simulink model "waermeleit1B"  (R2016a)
settings: Solver=ode45  StartTime=0.0  StopTime=2000  MaxStep=0.2  RelTol=1e-3
InitFcn:
  | init_waermeleit1
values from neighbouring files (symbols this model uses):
  dx = L/N    (= 0.2)    [init_waermeleit1.m]
  kappa = 1.1632e-04    (= 0.00011632)    [init_waermeleit1.m]
  T0 = 500    [init_waermeleit1.m]
  Tl = 300    [init_waermeleit1.m]
  Tr = 250    [init_waermeleit1.m]

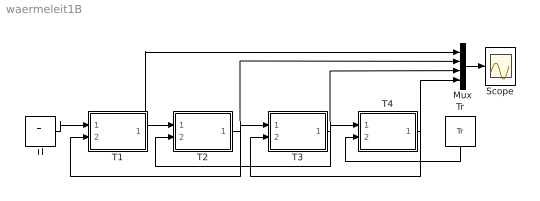
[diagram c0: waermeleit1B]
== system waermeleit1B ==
  Mux : Mux
  Scope : Scope
  T1 : Subsystem
  T2 : Subsystem
  T3 : Subsystem
  T4 : Subsystem
  Tl : Constant  Value=Tl
  Tr : Constant  Value=Tr
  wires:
  T1/1(T) -> Mux/1, T2/1(Tl)
  T2/1(T) -> T1/2(Tr), Mux/2, T3/1(Tl)
  T3/1(T) -> Mux/3, T4/1(Tl), T2/2(Tr)
  Tl/1 -> T1/1(Tl)
  T4/1(T) -> Mux/4, T3/2(Tr)
  Tr/1 -> T4/2(Tr)
  Mux/1 -> Scope/1

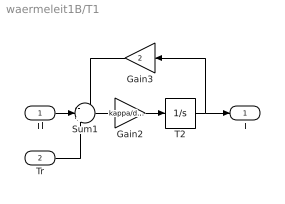
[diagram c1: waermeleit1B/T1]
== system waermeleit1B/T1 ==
  Tl : Inport
  Tr : Inport  Port=2
  Gain2 : Gain  Gain=kappa/dx^2
  Gain3 : Gain  Gain=2
  Sum1 : Sum  Inputs=-++
  T2 : Integrator  InitialCondition=T0
  T : Outport
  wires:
  Gain2/1 -> T2/1
  Sum1/1 -> Gain2/1
  T2/1 -> Gain3/1, T/1
  Gain3/1 -> Sum1/1
  Tl/1 -> Sum1/2
  Tr/1 -> Sum1/3

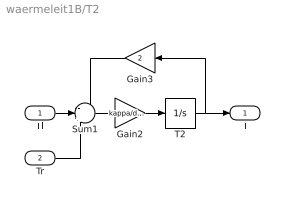
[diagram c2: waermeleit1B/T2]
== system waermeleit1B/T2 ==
  Tl : Inport
  Tr : Inport  Port=2
  Gain2 : Gain  Gain=kappa/dx^2
  Gain3 : Gain  Gain=2
  Sum1 : Sum  Inputs=-++
  T2 : Integrator  InitialCondition=T0
  T : Outport
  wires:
  Gain2/1 -> T2/1
  Sum1/1 -> Gain2/1
  T2/1 -> Gain3/1, T/1
  Gain3/1 -> Sum1/1
  Tl/1 -> Sum1/2
  Tr/1 -> Sum1/3

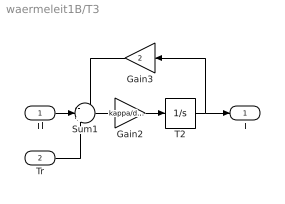
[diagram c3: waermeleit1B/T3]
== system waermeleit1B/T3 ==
  Tl : Inport
  Tr : Inport  Port=2
  Gain2 : Gain  Gain=kappa/dx^2
  Gain3 : Gain  Gain=2
  Sum1 : Sum  Inputs=-++
  T2 : Integrator  InitialCondition=T0
  T : Outport
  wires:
  Gain2/1 -> T2/1
  Sum1/1 -> Gain2/1
  T2/1 -> Gain3/1, T/1
  Gain3/1 -> Sum1/1
  Tl/1 -> Sum1/2
  Tr/1 -> Sum1/3

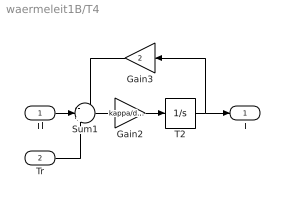
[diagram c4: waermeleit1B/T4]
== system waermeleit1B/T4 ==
  Tl : Inport
  Tr : Inport  Port=2
  Gain2 : Gain  Gain=kappa/dx^2
  Gain3 : Gain  Gain=2
  Sum1 : Sum  Inputs=-++
  T2 : Integrator  InitialCondition=T0
  T : Outport
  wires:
  Gain2/1 -> T2/1
  Sum1/1 -> Gain2/1
  T2/1 -> Gain3/1, T/1
  Gain3/1 -> Sum1/1
  Tl/1 -> Sum1/2
  Tr/1 -> Sum1/3
